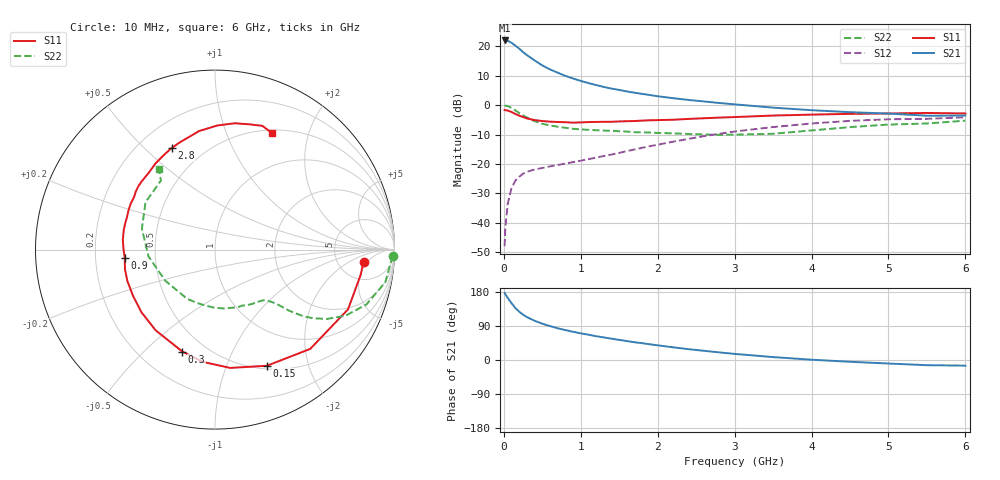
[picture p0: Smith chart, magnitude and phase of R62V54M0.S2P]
! SIEMENS Small Signal Semiconductors
! BFR193
! Si NPN RF Bipolar Junction Transistor in SOT23
! VCE = 2.5 V  IC = 4 mA
! Common Emitter S-Parameters:  May  1996
# GHz  S  MA  R  50
!  f  S11  S21  S12  S22
! GHz  MAG  ANG  MAG  ANG  MAG  ANG  MAG  ANG
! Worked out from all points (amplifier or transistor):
!   36 points, 10 MHz to 6 GHz, reference 50 ohm
!   highest |S21| = 22.0 dB at 10 MHz (marker M1)
!   |S21| within 3 dB of that: start of sweep to 208.8 MHz
!   unconditionally stable (mu >= 1): 941.4 MHz to 2.026 GHz
!   at 250 MHz: K = 0.37, MSG = 20.7 dB, |S12| = -23.3 dB
!   at 1.4 GHz: K = 1.08, MAG = 9.5 dB, |S12| = -16.8 dB
!   at 6 GHz: K = 0.97, MSG = 0.3 dB, |S12| = -4.1 dB
!   S11 on the Smith chart (normalised r, x): 10 MHz: 8.91, -4.07; 150 MHz: 0.54, -1.40; 300 MHz: 0.37, -0.66; 900 MHz: 0.33, -0.04; 2.8 GHz: 0.33, +0.61; 6 GHz: 0.54, +1.47
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0.01  0.8304 -4.9  12.63 177.1  0.004 90.6  0.9933 -2.1
0.02  0.8238 -9.8  12.61 173.5  0.0086 85.5  0.9814 -4.3
0.05  0.8125 -24.2  12.54 164.1  0.0208 78.3  0.9665 -10.8
0.1  0.7665 -46.2  11.5 150.0  0.0389 67.5  0.8974 -19.9
0.15  0.7089 -65.9  10.32 137.1  0.0521 59.0  0.8158 -26.8
0.2  0.6646 -82.7  9.158 127.5  0.0608 53.3  0.735 -31.7
0.25  0.6292 -96.2  7.992 119.6  0.0684 49.4  0.6687 -34.9
0.3  0.5963 -107.8  7.108 113.2  0.0737 46.6  0.6181 -37.0
0.4  0.5582 -126.3  5.778 103.5  0.0806 44.0  0.5352 -39.5
0.5  0.5382 -139.6  4.748 95.7  0.0854 43.6  0.4828 -40.7
0.6  0.5245 -150.6  4.065 89.4  0.0912 43.9  0.4532 -41.6
0.7  0.5186 -160.3  3.569 83.8  0.0963 45.2  0.4307 -42.7
0.9  0.505 -174.6  2.847 74.5  0.1077 48.8  0.3965 -45.2
1.1  0.5164 173.9  2.379 66.7  0.1208 52.2  0.3811 -49.0
1.3  0.5213 163.8  2.044 59.6  0.1367 54.9  0.3701 -53.0
1.6  0.5347 151.5  1.713 49.9  0.1655 57.8  0.3558 -61.1
2.2  0.5658 130.5  1.317 33.5  0.2396 57.8  0.3321 -81.1
2.8  0.6151 113.2  1.091 20.1  0.3263 52.1  0.3136 -108.7
3.5  0.6666 97.6  0.909 7.7  0.4252 40.9  0.3268 -147.9
4.5  0.7124 81.1  0.761 -4.7  0.5416 23.3  0.4238 164.0
5.5  0.7382 69.1  0.663 -13.7  0.5867 5.7  0.4884 128.1
6  0.7229 63.8  0.668 -14.9  0.6238 0.6  0.5461 124.9
